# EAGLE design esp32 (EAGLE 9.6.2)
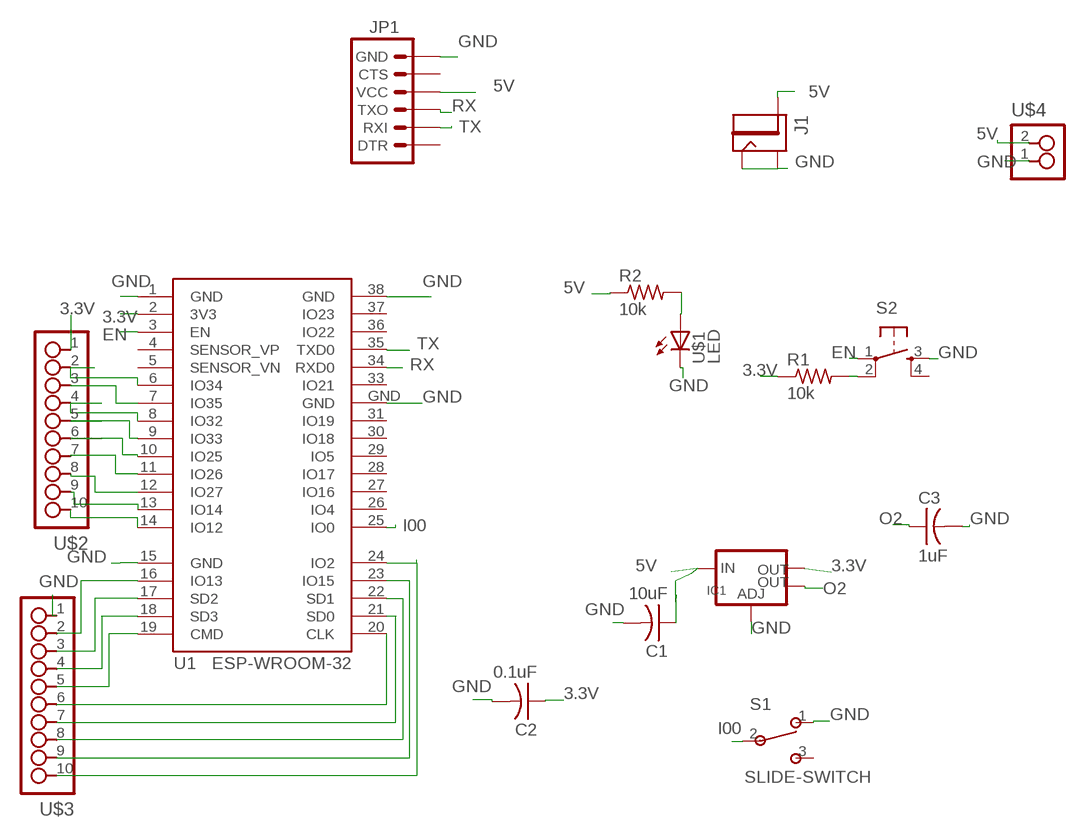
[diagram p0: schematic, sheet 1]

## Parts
C1  10uF  CAP-US1206  [C1206]
C2  0.1uF  CAP-US1206  [C1206]
C3  1uF  CAP-US1206  [C1206]
IC1  V_REG_LM1117SOT223  [SOT223]
J1  JACK2.1MM  [JACK_2.1MM]
JP1  FTDI_CONNECTORSMD  [1X06]
R1  10k  RES-US1206  [R1206]
R2  10k  RES-US1206  [R1206]
S1  SLIDE-SWITCH  [AYZ0102AGRLC]
S2  6MM_SWITCH6MM_SWITCH  [6MM_SWITCH]
U1  ESP-WROOM-32  [ESP-WROOM-32]
U$1  LED  [LED1206]
U$2  10_PIN_HEADERHEADER  [SMT_PINS_10]
U$3  10_PIN_HEADERHEADER  [SMT_PINS_10]
U$4  2_PIN_HEADERHEADER  [SMT_PINS_2]

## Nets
3.3V: C2.1 IC1.2(OUT) R1.1 U1.2(3V3) U$2.1
5V: C1.1 IC1.3(IN) J1.PIN JP1.4(VCC) R2.1 U$4.2
EN: S2.1(P) U1.3(EN)
GND: C1.2 C2.2 C3.2 IC1.1(ADJ) J1.CONTACT J1.SHUNT JP1.6(GND) S1.1 S2.3(S) U1.1(GND) U1.15(GND) U1.38(GND) U1.GND U$1.2(C) U$3.1 U$4.1
I00: S1.2 U1.25(IO0)
N$1: R1.2 S2.2(P1)
N$2: R2.2 U$1.1(A)
N$3: U1.6(IO34) U$2.2
N$4: U1.12(IO27) U$2.8
N$5: U1.7(IO35) U$2.3
N$6: U1.8(IO32) U$2.4
N$7: U1.9(IO33) U$2.5
N$8: U1.10(IO25) U$2.6
N$9: U1.11(IO26) U$2.7
N$10: U1.13(IO14) U$2.9
N$11: U1.14(IO12) U$2.10
N$12: U1.16(IO13) U$3.2
N$13: U1.17(SD2) U$3.3
N$14: U1.18(SD3) U$3.4
N$15: U1.19(CMD) U$3.5
N$16: U1.20(CLK) U$3.6
N$17: U1.21(SD0) U$3.7
N$18: U1.22(SD1) U$3.8
N$19: U1.23(IO15) U$3.9
N$20: U1.24(IO2) U$3.10
O2: C3.1 IC1.4(OUT)
RX: JP1.3(TXO) U1.34(RXD0)
TX: JP1.2(RXI) U1.35(TXD0)
Unconnected: JP1.1(DTR) JP1.5(CTS) S1.3 S2.4(S1) U1.4(SENSOR_VP) U1.5(SENSOR_VN) U1.26(IO4) U1.27(IO16) U1.28(IO17) U1.29(IO5) U1.30(IO18) U1.31(IO19) U1.33(IO21) U1.36(IO22) U1.37(IO23)

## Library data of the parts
C1-C3 = fab:CAP-US
IC1 = fab:V_REG_LM1117: Voltage Regulator LM1117 Standard adjustable voltage regulator but in SMD form. Spark Fun Electronics SKU : COM-00595; PROD_ID: VREG-08170
J1 = fablab:JACK
JP1 = fablab:FTDI_CONNECTOR: FTDI connector smd
R1 R2 = fab:RES-US: Resistor (US Symbol)
S1 = fab:SLIDE-SWITCH: SMD slide-switch AYZ0102AGRLC as found in the fablab inventory. Includes the mounting holes. Made by Zaerc.
S2 = fab:6MM_SWITCH: OMRON SWITCH
U1 = esp32:ESP-WROOM-32: Espressif Systems ESP-WROOM-32
U$1 = fab:LED: LED
U$2 U$3 = fablab:10_PIN_HEADER
U$4 = fablab:2_PIN_HEADER: 2 SMT pin pads

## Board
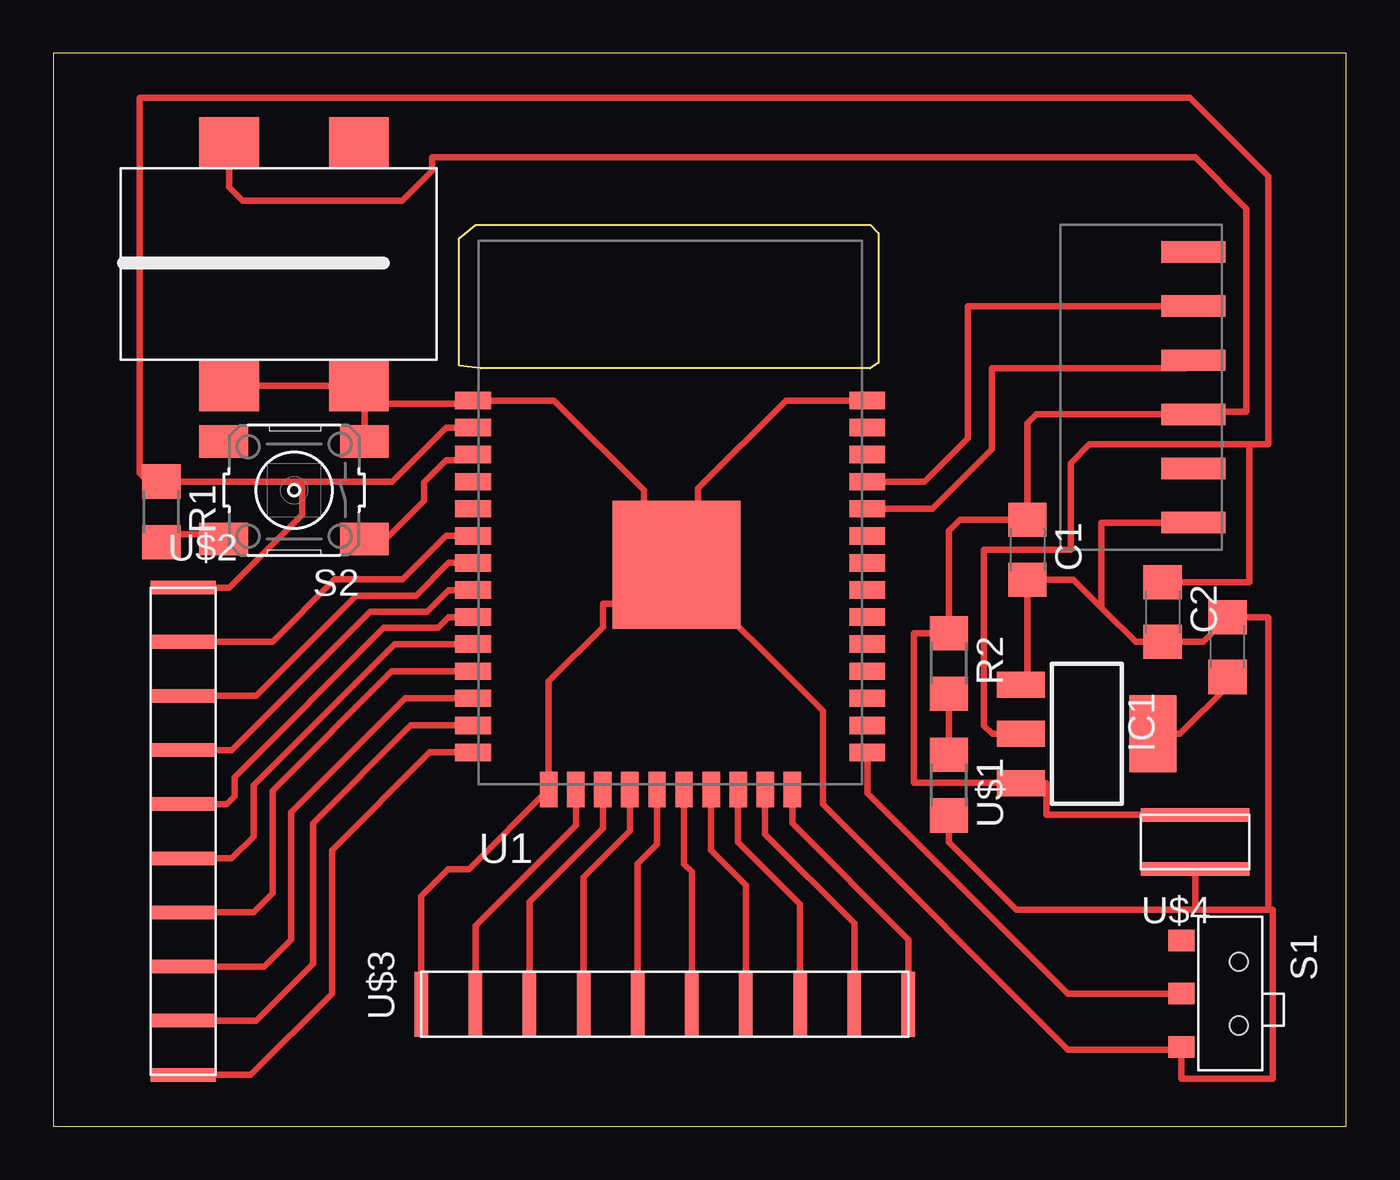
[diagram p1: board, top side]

Size 60.69 x 50.34 mm. Coordinates in mm from the lower left corner, seen from the top.
Outline: 0,0 60.69,0 60.69,50.34 0,50.34 0,0
Outline: 19.81,42.29 38.35,42.29 38.73,41.91 38.73,35.81 38.35,35.56 20.07,35.56 19.05,35.69 19.05,41.66 19.81,42.29
Copper layers (1*16): Top 0.035mm / dielectric 1.5mm / Bottom 0.035mm
Design rules "default": minimum track width 6mil, minimum drill 0.35mm, track to track 6mil, track to pad 6mil, pad to pad 6mil, via to via 6mil, smd to smd 6mil, copper to edge 40mil, drill to drill 6mil, minimum pad ring 10mil, minimum via ring 8mil, stop-mask expansion 4mil, vias tented up to drill 0mil, thermal gap 10mil

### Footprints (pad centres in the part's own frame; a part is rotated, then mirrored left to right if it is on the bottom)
C1206 = smd 1.6 x 1.8: 1 -1.4,0; 2 1.4,0
SOT223 = smd 1.219 x 2.235: 1 -2.311,-3.099; 2 0,-3.099; 3 2.311,-3.099 | smd 3.6 x 2.2: 4 0,3.099
JACK_2.1MM = smd 2.388 x 2.794: CONTACT 5.766,-2.413; PIN -5.639,-2.413; PIN1 -5.639,3.683; SHUNT 5.766,3.683
1X06 = smd 1 x 3: 1 -6.35,5; 2 -3.81,5; 3 -1.27,5; 4 1.27,5; 5 3.81,5; 6 6.35,5
R1206 = smd 1.6 x 1.803: 1 -1.422,0; 2 1.422,0
AYZ0102AGRLC = smd 1 x 1.2: 1 2.5,-2.3; 2 0,-2.3; 3 -2.5,-2.3 | hole 0.85: -1.5,0.4; 1.5,0.4
6MM_SWITCH = smd 2.286 x 1.524: 1 -3.302,2.286; 2 3.302,2.286; 3 -3.302,-2.286; 4 3.302,-2.286
ESP-WROOM-32 = smd 1.676 x 0.813: 1 -9.25,7; 2 -9.25,5.73; 3 -9.25,4.46; 4 -9.25,3.19; 5 -9.25,1.92; 6 -9.25,0.65; 7 -9.25,-0.62; 8 -9.25,-1.89; 9 -9.25,-3.16; 10 -9.25,-4.43; 11 -9.25,-5.7; 12 -9.25,-6.97; 13 -9.25,-8.24; 14 -9.25,-9.51; 25 9.25,-9.51; 26 9.25,-8.24; 27 9.25,-6.97; 28 9.25,-5.7; 29 9.25,-4.43; 30 9.25,-3.16; 31 9.25,-1.89; 32 9.25,-0.62; 33 9.25,0.65; 34 9.25,1.92; 35 9.25,3.19; 36 9.25,4.46; 37 9.25,5.73; 38 9.25,7 | smd 0.813 x 1.676: 15 -5.7,-11.25; 16 -4.43,-11.25; 17 -3.16,-11.25; 18 -1.89,-11.25; 19 -0.62,-11.25; 20 0.65,-11.25; 21 1.92,-11.25; 22 3.19,-11.25; 23 4.46,-11.25; 24 5.73,-11.25 | smd 6 x 6: GND 0.3,-0.7
LED1206 = smd 1.6 x 1.803: 1 -1.422,0; 2 1.422,0
SMT_PINS_10 = smd 3.048 x 0.635: 1 0,0; 2 0,2.54; 3 0,5.08; 4 0,7.62; 5 0,10.16; 6 0,12.7; 7 0,15.24; 8 0,17.78; 9 0,20.32; 10 0,22.86
SMT_PINS_2 = smd 5.08 x 0.635: 1 0,0; 2 0,2.54

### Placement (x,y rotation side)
C1  45.72,27.05 270 top
C2  52.07,24.13 270 top
C3  55.12,22.48 90 top
IC1  48.51,18.42 270 top
J1  10.67,40.51 270 top
JP1  48.51,34.67 270 top
R1  5.08,28.83 270 top
R2  42.04,21.72 270 top
S1  55.24,6.22 270 top
S2  11.3,29.85 180 top
U1  28.96,27.05 0 top
U$1  42.04,16 270 top
U$2  6.1,25.27 180 top
U$3  17.27,5.71 270 top
U$4  53.59,12.07 0 top

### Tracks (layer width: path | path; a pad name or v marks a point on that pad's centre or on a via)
3.3V
  Top 0.305: U1.2 18.44,32.78 15.91,30.25 11.68,30.25 | 11.68,30.25 R1.1 4.44,30.25 4.06,30.63 4.06,48.26 53.34,48.26 57.02,44.58 57.02,32 56.13,32 | 56.13,32 48.64,32 47.75,31.11 47.75,27.05 43.69,27.05 43.69,18.8 44.07,18.42 IC1.2 | 56.13,32 56.13,25.53 C2.1 | 11.68,30.25 11.68,28.7 8.25,25.27 U$2.1
5V
  Top 0.305: J1.PIN 8.25,44.07 8.89,43.43 16.38,43.43 17.78,44.83 17.78,45.47 53.59,45.47 56.01,43.05 56.01,33.53 53.51,33.53 JP1.4 46.15,33.4 45.72,32.97 C1.1 42.55,28.45 42.04,27.94 R2.1 40.39,23.14 40.39,16.13 45.39,16.13 IC1.3 46.61,16.1 46.61,14.61 U$4.2
EN
  Top 0.305: U1.3 19.45,31.26 18.44,31.26 17.4,30.22 17.4,29.34 15.62,27.56 S2.1
GND
  Top 0.152: 49.2,24.33 49.34,24.19
  Top 0.305: U1.GND 29.26,26.86 27.73,28.38 27.73,29.83 23.52,34.05 U1.1 arc-90 19.56,33.91 14.61,33.91 S2.3 14.61,34.49 J1.SHUNT J1.CONTACT | U1.GND 30.27,27.37 30.27,29.93 34.4,34.05 U1.38 | U1.GND 29.26,24.51 25.8,24.51 25.8,23.42 23.26,20.88 U1.15 19.52,12.07 18.54,12.07 17.27,10.79 U$3.1 | U1.GND 36.11,19.49 36.11,15.11 47.62,3.6 52.82,3.6 S1.1 52.95,2.22 57.24,2.22 57.24,10.16 57.02,10.16 | JP1.6 49.2,28.32 49.2,24.33 | IC1.1 45.72,21.03 C1.2 47.88,25.65 49.34,24.19 50.8,22.73 C2.2 53.97,22.73 C3.2 57.02,23.88 57.02,10.16 | U$1.2 42.04,13.33 45.21,10.16 53.59,10.16 | 57.02,10.16 53.85,10.16 53.59,10.16 | U$4.1 53.59,10.16
I00
  Top 0.305: S1.2 47.61,6.22 38.21,15.63 U1.25
N$1
  Top 0.305: S2.2 7.77,27.79 5.46,27.79 R1.2
N$2
  Top 0.305: R2.2 U$1.1
N$3
  Top 0.305: U1.6 18.44,27.7 16.39,25.65 13.21,25.65 10.29,22.73 U$2.2
N$4
  Top 0.305: U1.12 16.53,20.08 11.18,14.73 11.18,8.76 9.91,7.49 U$2.8
N$5
  Top 0.305: U1.7 18.56,26.43 17.02,24.89 14.22,24.89 9.53,20.19 U$2.3
N$6
  Top 0.305: U1.8 18.56,25.16 17.55,24.14 14.87,24.14 8.38,17.65 U$2.4
N$7
  Top 0.305: U1.9 18.56,23.89 18.05,23.38 15.51,23.38 8.51,16.38 8.51,15.49 8.13,15.11 U$2.5
N$8
  Top 0.305: U1.10 16.02,22.62 9.4,16 9.4,13.59 8.38,12.57 U$2.6
N$9
  Top 0.305: U1.11 15.89,21.35 10.29,15.75 10.29,10.92 9.4,10.03 U$2.7
N$10
  Top 0.305: U1.13 16.78,18.81 12.19,14.22 12.19,7.62 9.53,4.95 U$2.9
N$11
  Top 0.305: U1.14 17.67,17.54 13.08,12.95 13.08,6.22 9.27,2.41 U$2.10
N$12
  Top 0.305: U1.16 24.53,14.11 19.81,9.4 U$3.2
N$13
  Top 0.305: U1.17 25.8,13.99 22.35,10.54 U$3.3
N$14
  Top 0.305: U1.18 27.07,13.86 24.89,11.68 U$3.4
N$15
  Top 0.305: U1.19 28.34,13.22 27.43,12.32 U$3.5
N$16
  Top 0.305: U1.20 29.61,12.3 29.97,11.94 U$3.6
N$17
  Top 0.305: U1.21 30.88,12.94 32.51,11.3 U$3.7
N$18
  Top 0.305: U1.22 32.15,13.32 35.05,10.41 U$3.8
N$19
  Top 0.305: U1.23 33.42,13.7 37.59,9.53 U$3.9
N$20
  Top 0.305: U1.24 34.69,14.21 40.13,8.76 U$3.10
O2
  Top 0.305: C3.1 55.12,20.65 52.88,18.42 IC1.4
RX
  Top 0.305: JP1.3 53.13,35.56 44.05,35.56 44.05,31.76 41.25,28.97 U1.34
TX
  Top 0.305: JP1.2 42.93,38.48 42.93,32.27 40.89,30.24 U1.35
